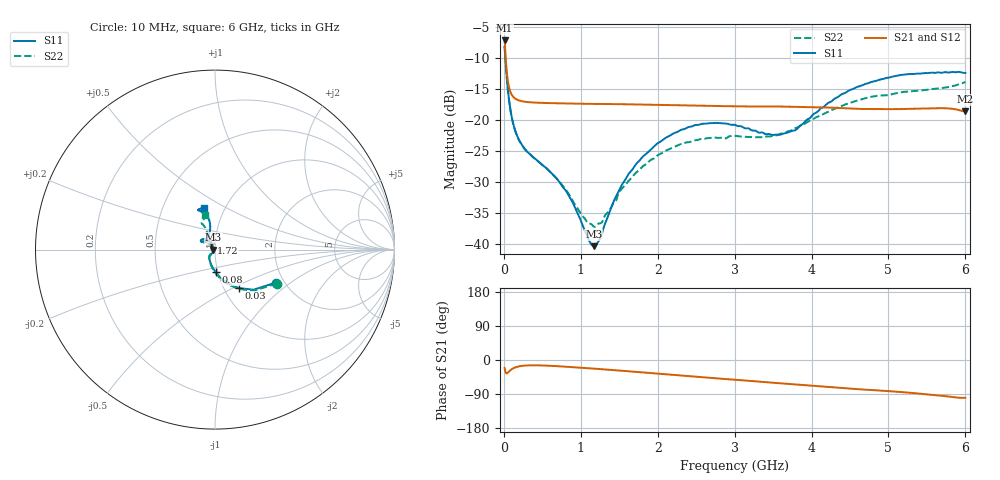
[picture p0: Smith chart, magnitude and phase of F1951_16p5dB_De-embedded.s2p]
! Integrated Device Technology
! Corporate Headquarters
! 6024 Silver Creek Valley Road
! San Jose, CA 95138  USA
! Phone:  1-408-284-8200
! Toll Free:  1-800-223-1366
! Webpage:  http://www.idt.com/
! Timing and RF Division
! 515 Groton Road, Suite 102
! Westford, MA 01886-6024
! Device:  F1951
! Description: 6-bit 0.5 dB Digital Step Attenuator
! Frequency:  100.0 -  4000.00 MHz
! Package:  4x4 mm Thin QFN Plastic Package: 24 pin
! Ports:  2 RF, 6 DC
!  Pin  1  = NC
!  Pin  2  = RF1  =  Port 1
!  Pin  3  = GND
!  Pin  4  = NC
!  Pin  5  = Serial Data Out (SDO)
!  Pin  6  = NC
!  Pin  7  = Reset Bar ( RSTb)
!  Pin  8  = Clock (CLK)
!  Pin  9  = Chip Select Bar (CSb)
!  Pin 10  = NC
!  Pin 11  = Serial Data In (SDI)
!  Pin 12  = NC
!  Pin 13  = NC
!  Pin 14  = VDD
!  Pin 15  = NC
!  Pin 16  = GND
!  Pin 17  = RF2  =  Port 2
!  Pin 18  = NC
!  Pin 19  = GND
!  Pin 20  = GND
!  Pin 21  = GND
!  Pin 22  = GND
!  Pin 23  = GND
!  Pin 24  = GND
! State:  33
! Atten State:  16.5 dB
! Voltage:  +3.30 Volts
! Current:  0.490 mA
! Data:  The device was measured on a F195X evaluation board which has
!  individual transmission lines to the RF pins.  Data was collected
!  de-embedded using a Automatic Fixture Removal [AFR] (Keysight Technologies).
!  The reference plane is the edge of the package pin.
! Misc:  Lot Code  1225BCA
!  Action Tracker AT0399
! Date Measured:  2018-09-13
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# GHz S dB R 50
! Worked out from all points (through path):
!   600 points, 10 MHz to 6 GHz, reference 50 ohm
!   highest |S21| = -7.22 dB at 10 MHz (marker M1); lowest = -18.6 dB at 6 GHz (marker M2)
!   group delay of S21, straight-line fit = 41.4 ps
!   lowest |S11| = -40.3 dB at 1.17 GHz (marker M3), VSWR 1.02, Z = 49 + j0.045 ohm
!   |S11| at or under -10 dB: 19.03 MHz to end of sweep
!   |S22| runs from -37.2 to -8.1 dB; largest |S21 - S12| = 0.00029
!   S11 on the Smith chart (normalised r, x): 10 MHz: 1.81, -0.78; 30 MHz: 1.17, -0.54; 80 MHz: 0.98, -0.25; 1.72 GHz: 0.95, +0.07; 6 GHz: 0.80, +0.39
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0.01  -8.27 -28.5  -7.22 -21.3  -7.22 -21.3  -8.11 -28.7
0.03  -11.99 -58.3  -11.06 -35.0  -11.06 -35.0  -11.93 -59.6
0.05  -14.90 -73.9  -13.52 -33.7  -13.53 -33.7  -14.90 -75.5
0.08  -17.94 -88.2  -15.31 -27.9  -15.31 -27.9  -17.98 -90.2
0.14  -21.45 -105.1  -16.51 -20.2  -16.51 -20.2  -21.47 -107.2
0.24  -24.11 -119.0  -17.01 -15.3  -17.01 -15.3  -24.19 -121.9
0.71  -29.81 -128.2  -17.34 -16.4  -17.33 -16.5  -29.79 -137.0
0.87  -32.77 -130.3  -17.38 -18.6  -17.38 -18.6  -32.46 -141.7
1.01  -36.55 -139.5  -17.42 -20.5  -17.42 -20.5  -35.31 -151.3
1.17  -40.35 177.3  -17.44 -22.7  -17.44 -22.7  -37.20 -178.3
1.27  -38.47 142.3  -17.44 -24.3  -17.45 -24.3  -36.57 160.8
1.52  -30.81 119.7  -17.49 -28.1  -17.49 -28.1  -31.29 134.8
1.72  -27.12 120.5  -17.52 -31.4  -17.52 -31.4  -28.50 131.1
2.01  -23.69 127.3  -17.59 -36.2  -17.59 -36.2  -25.62 133.8
2.49  -20.84 140.2  -17.70 -44.0  -17.70 -44.0  -23.28 141.9
3.01  -20.84 150.0  -17.82 -52.3  -17.82 -52.2  -22.57 145.6
3.59  -22.40 129.1  -17.86 -61.5  -17.86 -61.5  -22.26 127.8
3.79  -21.67 114.6  -17.92 -64.7  -17.93 -64.6  -21.34 121.0
4.01  -19.28 105.0  -17.95 -68.2  -17.95 -68.1  -19.98 115.6
4.49  -15.25 101.3  -18.16 -75.5  -18.16 -75.5  -17.30 114.1
5.01  -13.19 109.0  -18.29 -82.2  -18.29 -82.2  -16.01 116.7
6  -12.45 105.3  -18.65 -99.9  -18.65 -99.9  -13.92 105.4
